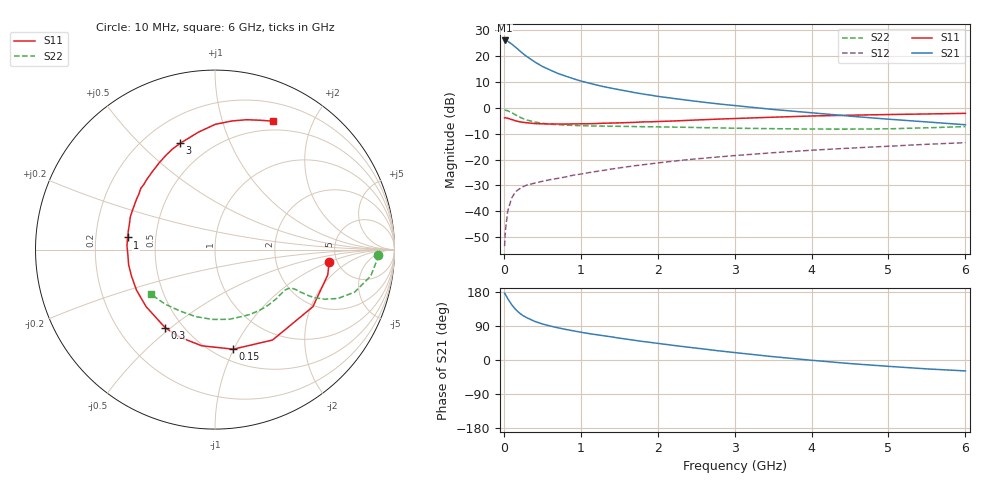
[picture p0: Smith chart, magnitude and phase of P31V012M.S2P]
! SIEMENS Small Signal Semiconductors
! BFP181
! Si NPN RF Bipolar Junction Transistor in SOT143
! VCE = 1 V  IC = 12 mA
! Common Emitter S-Parameters:  March  1996
# GHz  S  MA  R  50
!  f  S11  S21  S12  S22
! GHz  MAG  ANG  MAG  ANG  MAG  ANG  MAG  ANG
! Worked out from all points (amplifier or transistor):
!   36 points, 10 MHz to 6 GHz, reference 50 ohm
!   highest |S21| = 26.1 dB at 10 MHz (marker M1)
!   |S21| within 3 dB of that: start of sweep to 167 MHz
!   unconditionally stable (mu >= 1): start of sweep to 13.65 MHz; 435.1 MHz to end of sweep
!   at 250 MHz: K = 0.66, MSG = 25.8 dB, |S12| = -30.5 dB
!   at 1.4 GHz: K = 1.74, MAG = 10.6 dB, |S12| = -23.7 dB
!   at 6 GHz: K = 1.48, MAG = -0.6 dB, |S12| = -13.5 dB
!   S11 on the Smith chart (normalised r, x): 10 MHz: 4.30, -1.02; 150 MHz: 0.61, -1.00; 300 MHz: 0.40, -0.48; 1 GHz: 0.34, +0.06; 3 GHz: 0.34, +0.67; 6 GHz: 0.40, +1.48
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0.01  0.6402 -6.3  20.27 176.4  0.0021 76.0  0.9077 -1.8
0.02  0.6438 -12.7  20.2 173.1  0.0041 80.7  0.9035 -3.8
0.05  0.6314 -30.3  19.58 162.1  0.01 76.9  0.8809 -9.5
0.1  0.5972 -57.5  17.38 146.6  0.0177 63.6  0.8126 -17.0
0.15  0.5641 -79.6  15.09 134.1  0.0237 56.1  0.7365 -21.7
0.2  0.541 -97.8  13.02 124.4  0.0269 50.8  0.6716 -24.3
0.25  0.526 -112.0  11.23 117.0  0.0298 47.3  0.6196 -25.7
0.3  0.5158 -122.7  9.88 111.5  0.0321 45.3  0.5838 -26.2
0.4  0.4984 -140.4  7.797 102.0  0.0349 44.2  0.5337 -26.4
0.5  0.4923 -152.7  6.37 95.2  0.0379 42.8  0.5032 -26.3
0.6  0.4881 -162.2  5.439 89.8  0.0407 44.0  0.4847 -26.6
0.7  0.4886 -170.0  4.673 85.1  0.0432 45.1  0.4733 -27.0
1  0.492 172.1  3.326 73.4  0.0522 47.6  0.4532 -29.6
1.1  0.4943 167.3  3.045 69.9  0.0557 47.8  0.4492 -30.7
1.5  0.513 151.2  2.252 57.7  0.0689 48.8  0.44 -36.4
1.8  0.536 140.5  1.869 49.1  0.079 48.8  0.4335 -41.5
2.2  0.5578 128.6  1.531 38.7  0.0929 47.1  0.4253 -48.9
3  0.6231 108.2  1.112 19.6  0.1192 42.3  0.4044 -65.9
3.5  0.661 98.0  0.934 8.8  0.1357 39.0  0.3966 -78.3
4.5  0.7228 82.5  0.693 -9.4  0.1665 30.8  0.3886 -105.8
5.5  0.7639 70.6  0.535 -23.5  0.1976 22.9  0.4119 -132.6
6  0.7851 65.7  0.472 -28.8  0.2125 18.3  0.4348 -145.2
